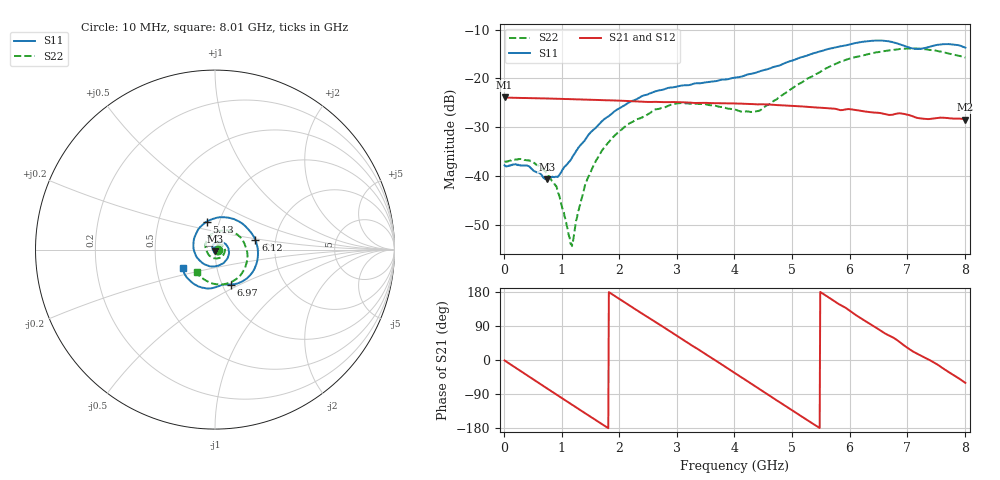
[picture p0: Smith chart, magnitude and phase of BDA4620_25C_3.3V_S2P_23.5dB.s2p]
!Agilent Technologies,E5071B,MY42404982,A.09.10
!Date: Wed May 06 08:53:54 2026
!Data & Calibration Information:
!Freq	S11:SOLT2(ON)	S21:SOLT2(ON)	S12:SOLT2(ON)	S22:SOLT2(ON)
# Hz S RI R 50
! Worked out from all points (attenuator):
!   801 points, 10 MHz to 8.01 GHz, reference 50 ohm
!   highest |S21| = -23.90 dB at 10 MHz (marker M1); lowest = -28.4 dB at 8.01 GHz (marker M2)
!   lowest |S11| = -40.6 dB at 740 MHz (marker M3), VSWR 1.02, Z = 49.9 - j0.925 ohm
!   |S11| at or under -10 dB: start of sweep to end of sweep
!   |S22| runs from -54.3 to -13.9 dB; largest |S21 - S12| = 0.00028
!   S11 on the Smith chart (normalised r, x): 10 MHz: 1.03, -0.00; 5.13 GHz: 0.87, +0.28; 6.12 GHz: 1.57, +0.18; 6.97 GHz: 1.10, -0.45; 8.01 GHz: 0.68, -0.14
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1e7  0.0129 -0.000785  0.0638 -0.00135  0.0639 -0.00136  0.014 -0.000441
4.4e8  0.00903 -0.00868  0.045 -0.044  0.045 -0.0441  0.0134 -0.00516
7.4e8  -0.00136 -0.00928  0.0169 -0.06  0.0169 -0.0601  0.00793 -0.00728
9.3e8  -0.00817 -0.00543  -0.00338 -0.0618  -0.00349 -0.0619  0.00349 -0.00635
1.16e9  -0.0141 0.00454  -0.0269 -0.0552  -0.027 -0.0552  -0.00159 -0.00122
1.2e9  -0.0147 0.00671  -0.0306 -0.0531  -0.0306 -0.0532  -0.00219 -2.42e-05
1.35e9  -0.015 0.0154  -0.0429 -0.0432  -0.0429 -0.0433  -0.00377 0.00463
1.53e9  -0.0111 0.0268  -0.0536 -0.0279  -0.0537 -0.028  -0.00358 0.0114
1.77e9  0.00157 0.0393  -0.0597 -0.00416  -0.0597 -0.00418  0.000564 0.0207
2.15e9  0.0345 0.0439  -0.0491 0.0324  -0.0492 0.0325  0.0171 0.0295
2.68e9  0.075 0.00618  -0.00543 0.0572  -0.00538 0.0573  0.0446 0.0197
3.08e9  0.0705 -0.0465  0.0316 0.0475  0.0318 0.0475  0.0555 -0.0073
4.01e9  -0.067 -0.0771  0.0456 -0.0316  0.0456 -0.0317  -0.0106 -0.0468
4.43e9  -0.1179 -0.00195  0.0132 -0.0527  0.0131 -0.0528  -0.0453 -0.0118
5.13e9  -0.0473 0.1555  -0.0426 -0.0295  -0.0427 -0.0294  -0.0143 0.0873
5.35e9  0.0154 0.1786  -0.0494 -0.0115  -0.0495 -0.0115  0.0228 0.1025
5.69e9  0.1239 0.1616  -0.0463 0.0172  -0.0463 0.0171  0.0895 0.1017
6.12e9  0.2252 0.0531  -0.0218 0.0419  -0.0218 0.0421  0.1619 0.0382
6.68e9  0.1804 -0.1582  0.0181 0.0383  0.0181 0.0384  0.1706 -0.0909
6.97e9  0.0878 -0.1946  0.0349 0.0251  0.035 0.0252  0.1307 -0.1538
7.6e9  -0.0727 -0.2115  0.0374 -0.0135  0.0375 -0.0134  -0.0236 -0.1862
8.01e9  -0.1806 -0.1  0.0187 -0.0329  0.0189 -0.0331  -0.1025 -0.1271
